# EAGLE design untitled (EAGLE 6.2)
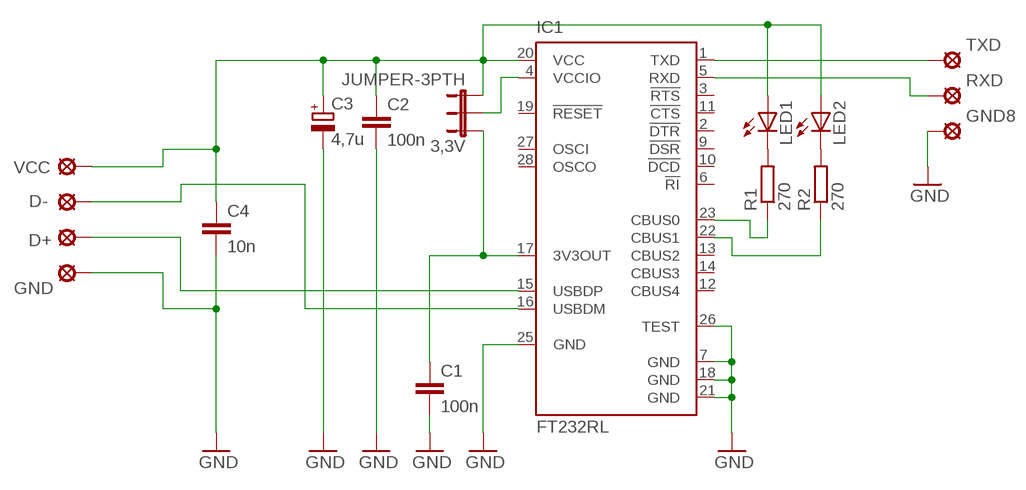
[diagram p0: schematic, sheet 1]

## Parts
3,3V  JUMPER-3PTH  [1X03]
C1  100n  C-EUC1210  [C1210]
C2  100n  C-EUC1210  [C1210]
C3  4,7u  CPOL-EU153CLV-0405  [153CLV-0405]
C4  10n  C-EUC1206  [C1206]
D+  LSP11  [LSP11]
D-  LSP11  [LSP11]
GND  LSP11  [LSP11]
GND8  LSP11  [LSP11]
IC1  FT232RL  [SSOP28]
LED1  LED-FKIT-1206  [FKIT-LED-1206]
LED2  LED-FKIT-1206  [FKIT-LED-1206]
R1  270  R-EU_R1206  [R1206]
R2  270  R-EU_R1206  [R1206]
RXD  LSP11  [LSP11]
TXD  LSP11  [LSP11]
VCC  LSP11  [LSP11]

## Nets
GND: C1.2 C2.2 C3.- C4.2 GND8.MP GND.MP IC1.7(GND) IC1.18(GND) IC1.21(GND) IC1.25(GND) IC1.26(TEST)
N$1: 3,3V.1 C1.1 IC1.17(3V3OUT)
N$2: D-.MP IC1.16(USBDM)
N$3: 3,3V.2 IC1.4(VCCIO)
N$4: IC1.1(TXD) TXD.MP
N$5: IC1.5(RXD) RXD.MP
N$6: D+.MP IC1.15(USBDP)
N$7: IC1.23(CBUS0) R1.1
N$8: IC1.22(CBUS1) R2.1
N$9: LED1.C R1.2
N$10: LED2.C R2.2
N$12: 3,3V.3 C2.1 C3.+ C4.1 IC1.20(VCC) LED1.A LED2.A VCC.MP
Unconnected: IC1.2(!DTR) IC1.3(!RTS) IC1.6(!RI) IC1.9(!DSR) IC1.10(!DCD) IC1.11(!CTS) IC1.12(CBUS4) IC1.13(CBUS2) IC1.14(CBUS3) IC1.19(!RESET) IC1.27(OSCI) IC1.28(OSCO)

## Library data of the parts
3,3V = SparkFun:JUMPER-3
C1 C2 C4 = rcl:C-EU: CAPACITOR, European symbol
C3 = rcl:CPOL-EU: POLARIZED CAPACITOR, European symbol
D+ D- GND GND8 RXD TXD VCC = solpad:LSP11: SOLDER PAD
IC1 = ftdichip:FT232R: Source: http://www.ftdichip.com/Documents/DataSheets/DS_FT232R_v104.pdf; MPN: FT232RL; OC_FARNELL: 1146032; OC_NEWARK: 91K9918
LED1 LED2 = SparkFun:LED: LEDs
R1 R2 = rcl:R-EU_: RESISTOR, European symbol

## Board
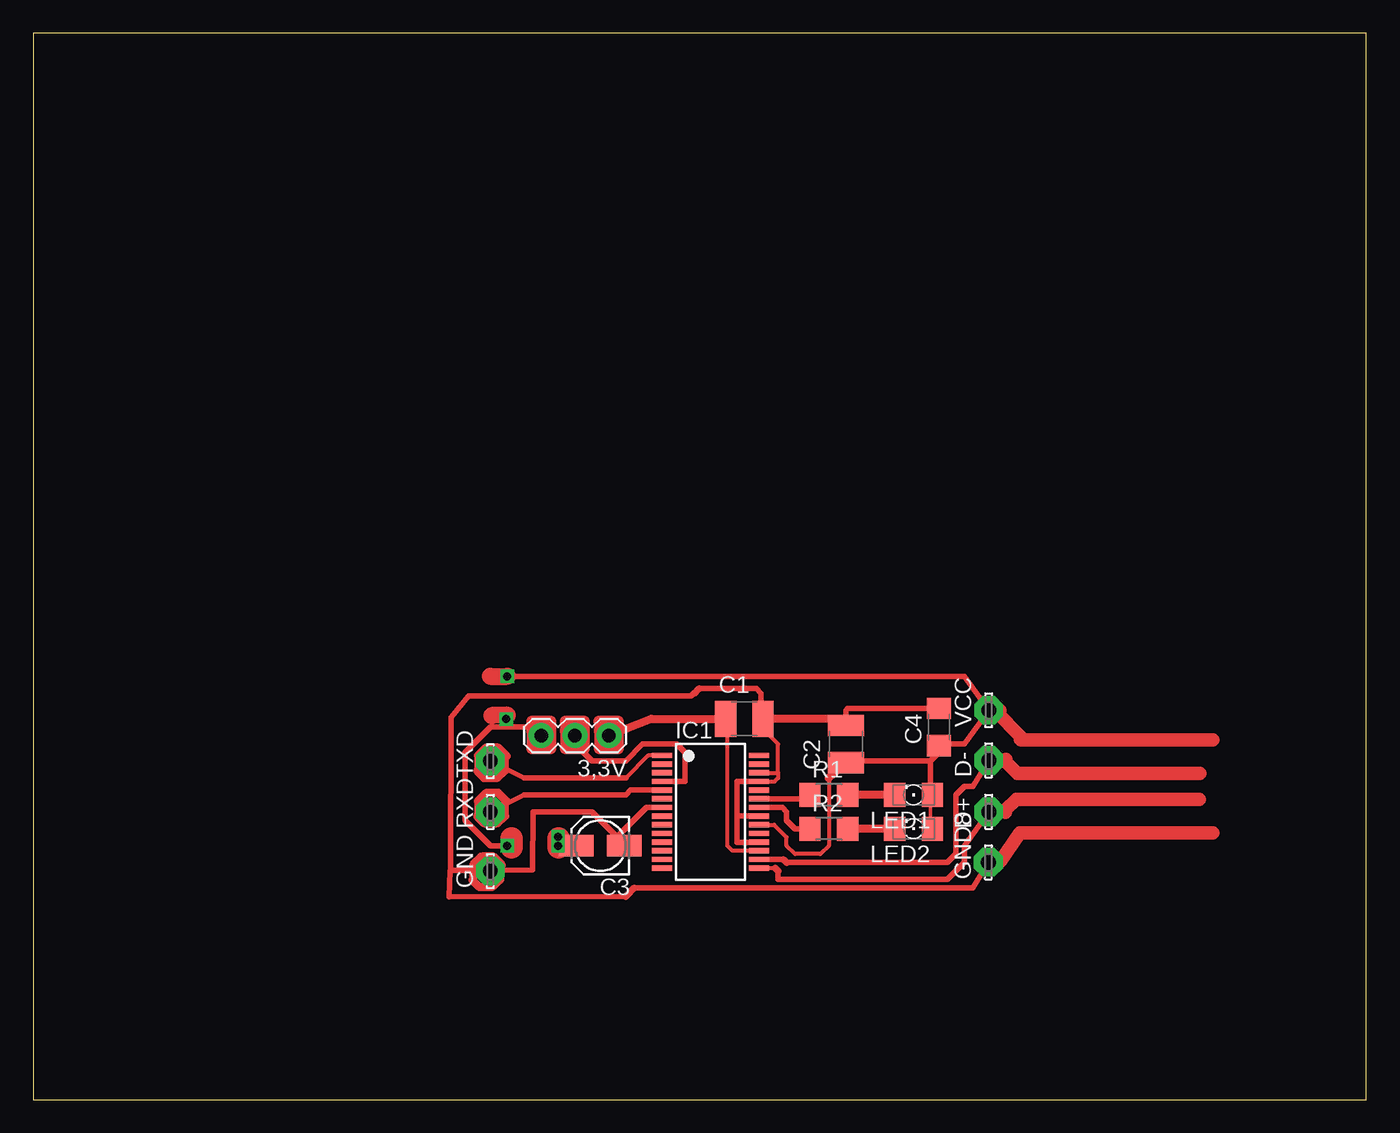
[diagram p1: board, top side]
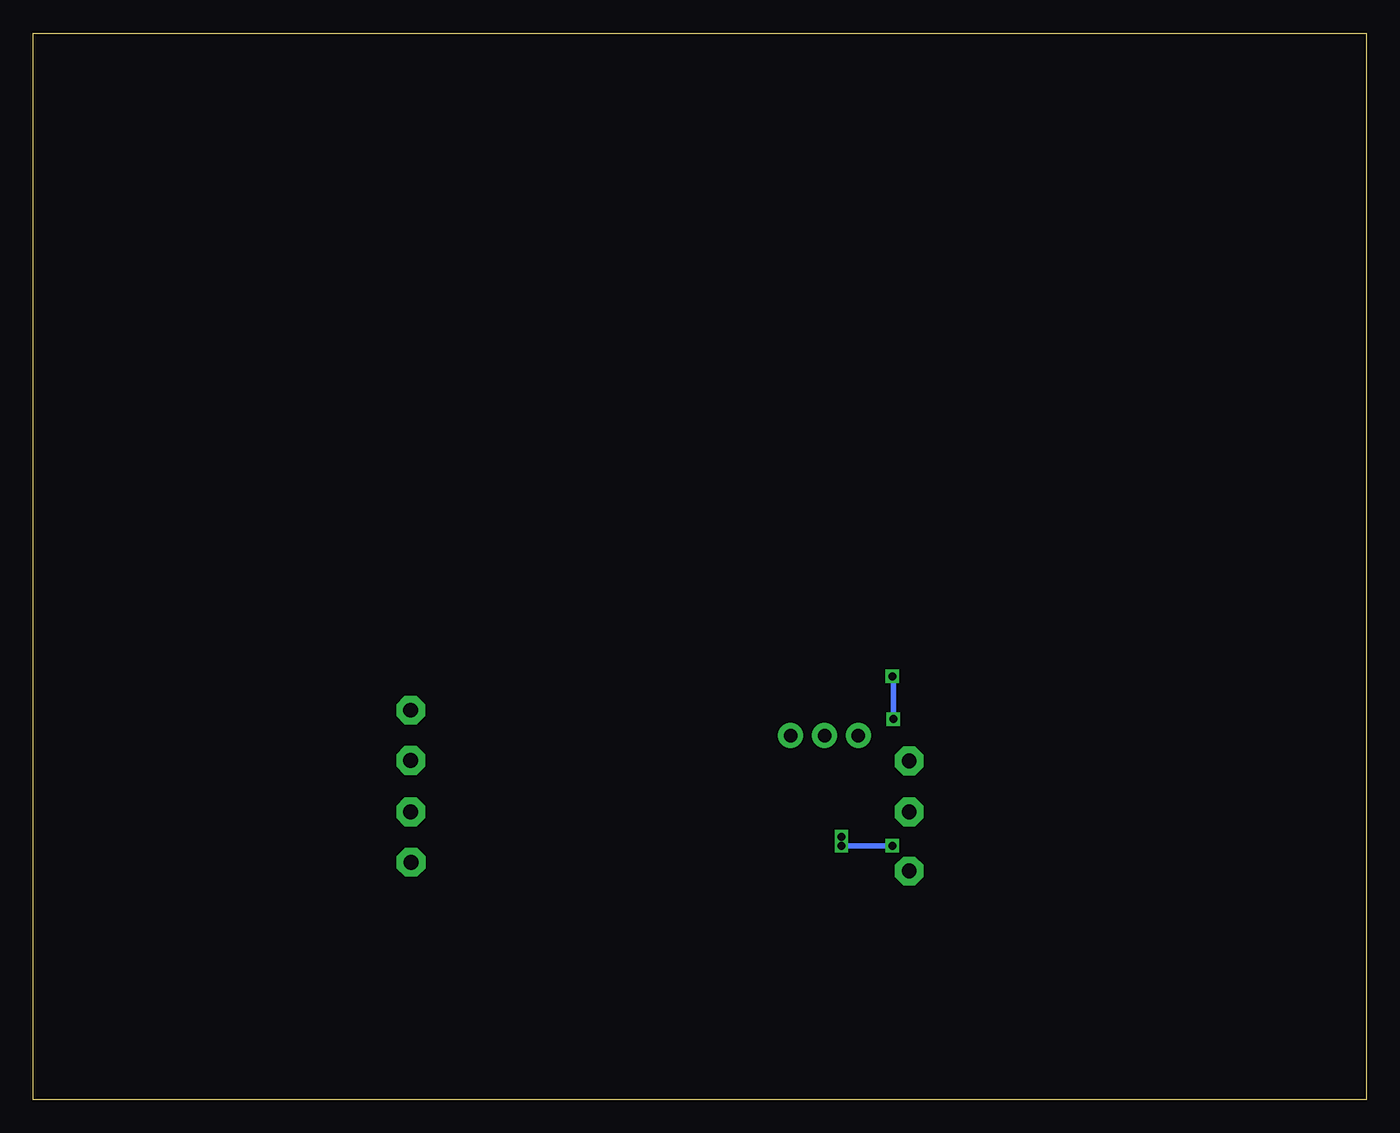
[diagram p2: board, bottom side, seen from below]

Size 100 x 80 mm. Coordinates in mm from the lower left corner, seen from the top.
Outline: 0,0 100,0 100,80 0,80 0,0
Copper layers (1*16): Top 0.035mm / dielectric 1.5mm / Bottom 0.035mm
Design rules: minimum track width 10mil, minimum drill 24mil, track to track 8mil, track to pad 8mil, pad to pad 8mil, via to via 8mil, smd to smd 8mil, copper to edge 40mil, drill to drill 8mil, minimum pad ring 10mil, minimum via ring 8mil, stop-mask expansion 4mil, vias tented up to drill 0mil, thermal gap 10mil

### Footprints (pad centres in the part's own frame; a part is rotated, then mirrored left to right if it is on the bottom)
1X03 = drill 1.016 pad 1.88: 1 0,0; 2 2.54,0; 3 5.08,0
C1210 = smd 1.6 x 2.7: 1 -1.4,0; 2 1.4,0
153CLV-0405 = smd 2.6 x 1.6: + 1.8,0; - -1.8,0
C1206 = smd 1.6 x 1.8: 1 -1.4,0; 2 1.4,0
LSP11 = drill 1.118 pad 2.159 octagon: MP 0,0
SSOP28 = smd 0.4 x 1.5: 1 -4.225,-3.625; 2 -3.575,-3.625; 3 -2.925,-3.625; 4 -2.275,-3.625; 5 -1.625,-3.625; 6 -0.975,-3.625; 7 -0.325,-3.625; 8 0.325,-3.625; 9 0.975,-3.625; 10 1.625,-3.625; 11 2.275,-3.625; 12 2.925,-3.625; 13 3.575,-3.625; 14 4.225,-3.625; 15 4.225,3.625; 16 3.575,3.625; 17 2.925,3.625; 18 2.275,3.625; 19 1.625,3.625; 20 0.975,3.625; 21 0.325,3.625; 22 -0.325,3.625; 23 -0.975,3.625; 24 -1.625,3.625; 25 -2.275,3.625; 26 -2.925,3.625; 27 -3.575,3.625; 28 -4.225,3.625
FKIT-LED-1206 = smd 1.6 x 1.803: A -1.422,0; C 1.422,0
R1206 = smd 1.6 x 1.803: 1 -1.422,0; 2 1.422,0

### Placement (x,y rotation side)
3,3V  43.18,27.3 180 top
C1  53.34,28.57 0 top
C2  60.96,26.67 90 top
C3  42.55,19.05 180 top
C4  67.94,27.94 90 top
D+  71.68,21.59 90 top
D-  71.68,25.45 90 top
GND  34.29,17.14 90 top
GND8  71.65,17.81 90 top
IC1  50.8,21.59 270 top
LED1  66.04,22.86 180 top
LED2  66.04,20.32 180 top
R1  59.69,22.86 0 top
R2  59.69,20.32 0 top
RXD  34.29,21.59 90 top
TXD  34.29,25.4 90 top
VCC  71.68,29.21 90 top

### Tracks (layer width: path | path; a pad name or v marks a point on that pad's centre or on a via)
GND
  Top 0.254: 43.76,19.69 C3.- | 60.96,28.57 C2.2 | 54.61,27.94 C1.2
  Top 0.305: IC1.25 55.62,23.86 55.88,24.13 55.88,24.52 | 55.88,24.52 55.88,26.67 54.61,27.94 | IC1.26 55.88,24.52
  Top 0.406: 45.09,15.88 70.48,15.88 GND8.MP | 44.45,15.24 31.19,15.21 31.27,17.14 31.77,17.2 | C2.2 60.96,29.21 61.09,29.34 C4.2 | IC1.7 45.99,21.91 43.76,19.69 43.76,19.74 41.91,21.59 37.49,21.57 37.44,17.22 34.31,17.2 | 34.31,17.2 GND.MP | 34.31,17.2 31.77,17.2 | IC1.25 52.78,23.86 52.78,21.27 | 52.78,21.27 52.78,19.3 54.42,19.3 IC1.18 | IC1.21 52.78,21.27 | 31.77,17.2 31.29,17.2 31.34,28.68 32.64,30.28 49.33,30.28 49.53,30.48 49.61,30.48 | 49.96,30.84 54.25,30.84 54.61,30.48 54.61,28.7 C1.2
  Top 0.508: 45.09,15.88 44.45,15.24 | 49.61,30.48 49.96,30.84
  Top 0.61: 60.96,28.57 C1.2
  Top 1.016: GND8.MP 72.47,17.78
N$1
  Top 0.254: 52.07,29.21 C1.1 52.07,27.94
  Top 0.305: IC1.17 52.45,18.66 52.07,19.05 52.07,27.94
  Top 0.61: C1.1 46.35,28.57 3,3V.1
N$2
  Top 0.406: IC1.16 56.28,18.02 | 56.52,17.78 57.15,17.78 68.58,17.78 69.22,18.41 69.22,22.86 69.85,23.5 70.48,23.5 D-.MP
  Top 0.508: 56.28,18.02 56.52,17.78
  Top 1.016: D-.MP 72.48,25.45
N$3
  Top 0.406: IC1.4 48.9,23.86 48.9,26.04 48.26,26.67 45.72,26.67 44.45,25.4 41.91,25.4 40.64,26.67 3,3V.2
N$4
  Top 0.305: IC1.1 46.13,25.82 44.45,24.13
  Top 0.406: 44.45,24.13 36.83,24.13 TXD.MP
N$5
  Top 0.406: IC1.5 44.8,23.21 44.45,22.86 36.83,22.86 RXD.MP
N$6
  Top 0.305: IC1.15 55.66,17.36
  Top 0.406: 55.88,17.14 55.88,16.51 68.58,16.51 69.85,17.78 69.85,19.05 D+.MP
  Top 0.508: 55.66,17.36 55.88,17.14
  Top 1.016: D+.MP 72.52,21.64
N$7
  Top 0.406: IC1.23 57.97,22.57 R1.1
N$8
  Top 0.406: IC1.22 56.19,21.91 56.52,21.59 56.52,20.95 57.15,20.32 R2.1
N$9
  Top 0.254: 60.96,22.86 R1.2 | 64.77,22.86 LED1.C
  Top 0.61: LED1.C R1.2
N$10
  Top 0.254: 60.96,20.32 R2.2 | 64.77,20.32 LED2.C
  Top 0.61: LED2.C R2.2
N$12  (via drill 0.6)
  Top 0.254: 60.96,25.4 C2.1 | LED2.A 67.31,20.32 67.31,22.86 LED1.A
  Top 0.305: 59.69,24.13 59.69,19.05 59.05,18.41 57.15,18.41 56.52,19.05 56.52,19.68 55.59,20.61 IC1.20
  Top 0.406: 67.31,25.4 60.96,25.4 | 67.31,22.86 67.31,25.4 | C3.+ v39.37,19.05 | v35.56,19.05 34.29,19.05 32.38,20.95 32.38,26.04 34.29,27.94 35.56,27.94 | 3,3V.3 37.47,27.94 35.56,27.94 | 67.31,25.4 67.94,26.04 C4.1 68.45,26.54 68.58,26.67 69.85,26.67 VCC.MP 69.85,31.75 v35.56,31.75 | 35.56,27.94 35.56,28.47 v35.48,28.55
  Top 0.61: C2.1 59.69,24.13
  Top 1.016: VCC.MP 72.52,29.21
  Top 1.27: 34.29,31.75 v35.56,31.75
  Bottom 0.406: v39.37,19.05 v35.56,19.05 | v35.48,28.55 35.48,31.67 v35.56,31.75
N$13
  Top 1.27: 35.56,28.85 34.42,28.8
N$14
  Top 1.676: 39.4,19.58 39.4,18.92 | 35.89,19.58 35.89,18.92
N$15
  Top 0.813: 37.41,27.61 37.41,26.34 38.84,26.34 38.84,28.37 37.39,28.37 37.41,27.71
N$16  (via drill 0.6)
  other vias: 39.37,19.71
N$17
  Top 1.016: 72.97,25.5 72.97,25.35 73.84,24.49 87.5,24.49
N$18
  Top 1.016: 72.95,21.54 72.95,21.72 73.76,22.53 87.48,22.53
N$19
  Top 1.016: 88.51,20 74,20 72.54,17.88
N$20
  Top 1.016: 88.49,26.98 74.14,26.98
N$21
  Top 1.016: 74.07,27.03 74.07,27.25 72.24,29.08
N$23
  Top 0.813: 42.47,27.61 42.47,26.34 43.89,26.34 43.89,28.37 42.44,28.37 42.47,27.71
N$24
  Top 0.813: 39.93,27.61 39.93,26.34 41.35,26.34 41.35,28.37 39.9,28.37 39.93,27.71
N$25
  Top 0.406: 33.66,18.24 33.63,18.21 33.58,18.21 | 32.99,16.59 32.94,16.54 32.94,16.46 | 34.39,15.95 34.42,15.98 34.49,15.98 | 34.95,16.43 35,16.43 35.05,16.48 | 35.05,17.48 35.13,17.55
  Top 0.61: 35.15,17.6 34.52,18.24 33.66,18.24 | 33.58,18.21 32.99,17.63 32.99,16.59 | 32.94,16.46 33.45,15.95 34.39,15.95 | 34.49,15.98 34.95,16.43 | 35.05,16.48 35.05,17.48
N$26
  Top 0.406: 34.01,23.01 33.98,22.99 33.93,22.99 | 33.35,21.36 33.3,21.31 33.3,21.23 | 34.75,20.73 34.77,20.75 34.85,20.75 | 35.31,21.21 35.36,21.21 35.41,21.26 | 35.41,22.25 35.48,22.33
  Top 0.61: 35.51,22.38 34.87,23.01 34.01,23.01 | 33.93,22.99 33.35,22.4 33.35,21.36 | 33.3,21.23 33.81,20.73 34.75,20.73 | 34.85,20.75 35.31,21.21 | 35.41,21.26 35.41,22.25
N$27
  Top 0.406: 34.01,26.42 33.98,26.39 33.93,26.39 | 33.35,24.77 33.3,24.71 33.3,24.64 | 34.75,24.13 34.77,24.16 34.85,24.16 | 35.31,24.61 35.36,24.61 35.41,24.66 | 35.41,25.65 35.48,25.73
  Top 0.61: 35.51,25.78 34.87,26.42 34.01,26.42 | 33.93,26.39 33.35,25.81 33.35,24.77 | 33.3,24.64 33.81,24.13 34.75,24.13 | 34.85,24.16 35.31,24.61 | 35.41,24.66 35.41,25.65

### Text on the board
Document: TX | 5V | 3,3V | TX | RX | RX | GND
